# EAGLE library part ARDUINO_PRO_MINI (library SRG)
Arduino Pro-Mini Made by Sparkfun Comes in 3.3 volt and 5 volt versions Note: A6 & A7 are analog in only
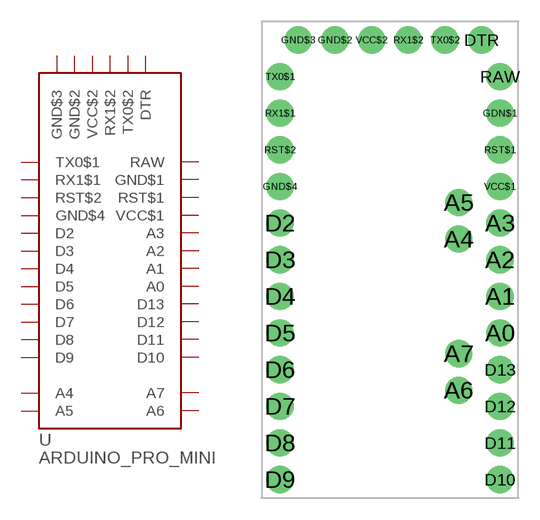
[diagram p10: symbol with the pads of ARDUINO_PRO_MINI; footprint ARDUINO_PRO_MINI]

Designator prefix -

## ARDUINO_PRO_MINI  [ARDUINO_PRO_MINI]
A0  A0
A1  A1
A2  A2
A3  A3
A4  A4
A5  A5
A6  A6  in
A7  A7  in
D2  D2
D3  D3
D4  D4
D5  D5
D6  D6
D7  D7
D8  D8
D9  D9
D10  D10
D11  D11
D12  D12
D13  D13
DTR  DTR  in
GDN$1  GND$1  pwr
GND$2  GND$2  pwr
GND$3  GND$3  pwr
GND$4  GND$4  pwr
RAW  RAW  pwr
RST$1  RST$1  in
RST$2  RST$2  in
RX1$1  RX1$1
RX1$2  RX1$2
TX0$1  TX0$1
TX0$2  TX0$2
VCC$1  VCC$1  pwr
VCC$2  VCC$2  pwr

## Footprint ARDUINO_PRO_MINI (pad centres in mm)
Arduino Pro-Mini Made by Sparkfun
drill 1.016 pad 1.88: A0 7.62,-5.08; A1 7.62,-2.54; A2 7.62,0; A3 7.62,2.54; A4 4.763,1.429; A5 4.763,3.969; A6 4.763,-9.049; A7 4.763,-6.509; D2 -7.62,2.54; D3 -7.62,0; D4 -7.62,-2.54; D5 -7.62,-5.08; D6 -7.62,-7.62; D7 -7.62,-10.16; D8 -7.62,-12.7; D9 -7.62,-15.24; D10 7.62,-15.24; D11 7.62,-12.7; D12 7.62,-10.16; D13 7.62,-7.62; DTR 6.35,15.24; GDN$1 7.62,10.16; GND$2 -3.81,15.24; GND$3 -6.35,15.24; GND$4 -7.62,5.08; RAW 7.62,12.7; RST$1 7.62,7.62; RST$2 -7.62,7.62; RX1$1 -7.62,10.16; RX1$2 1.27,15.24; TX0$1 -7.62,12.7; TX0$2 3.81,15.24; VCC$1 7.62,5.08; VCC$2 -1.27,15.24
